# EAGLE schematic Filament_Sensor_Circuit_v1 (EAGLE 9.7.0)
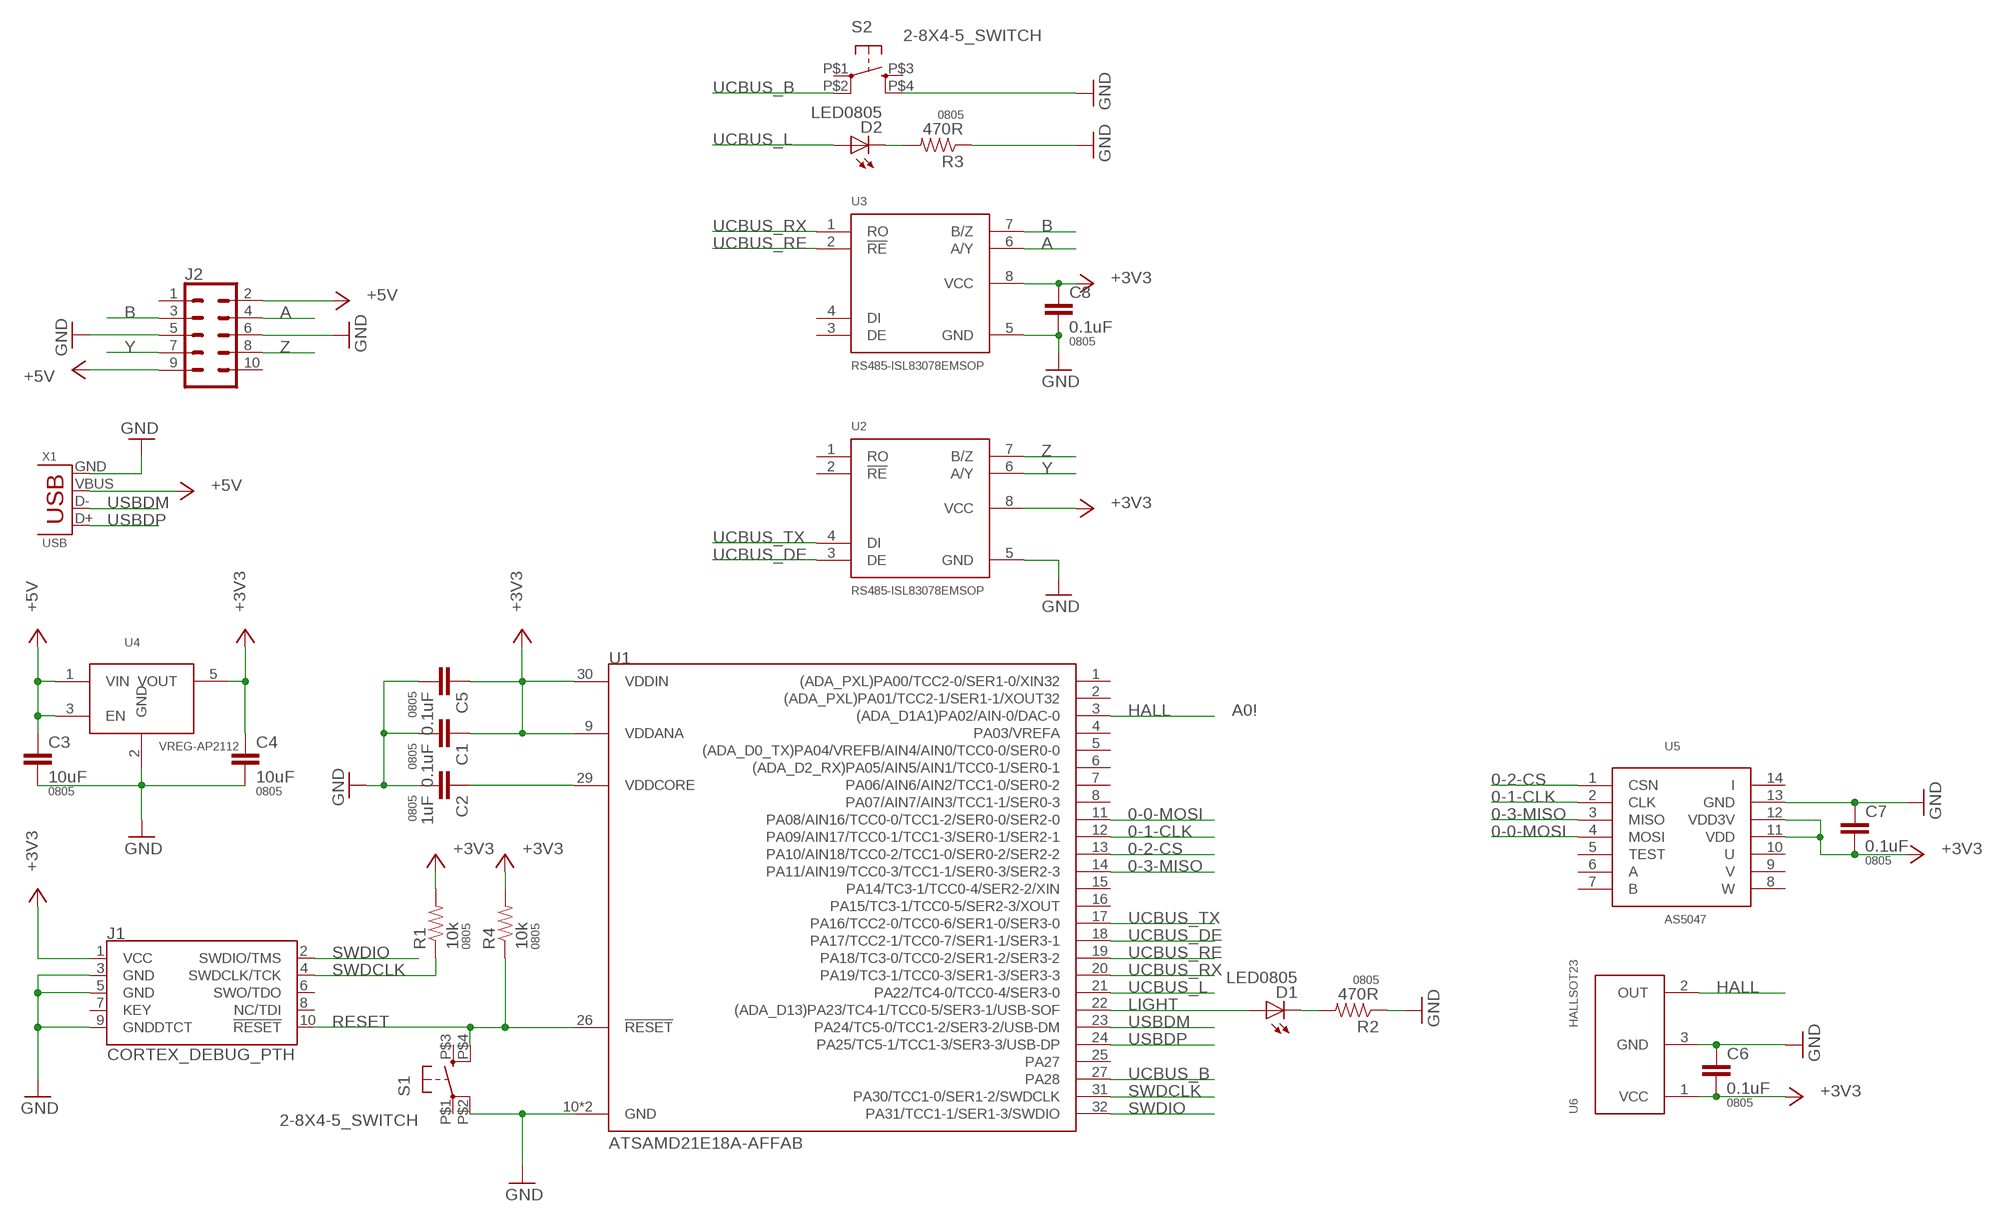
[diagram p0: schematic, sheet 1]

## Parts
C1  0.1uF  CAP0805  [0805]
C2  1uF  CAP0805  [0805]
C3  10uF  CAP0805  [0805]
C4  10uF  CAP0805  [0805]
C5  0.1uF  CAP0805  [0805]
C6  0.1uF  CAP0805  [0805]
C7  0.1uF  CAP0805  [0805]
C8  0.1uF  CAP0805  [0805]
D1  LED0805  [LED0805]
D2  LED0805  [LED0805]
J1  CORTEX_DEBUG_PTH  [2X5-PTH-1.27MM]
J2  CONN_05X2SHD_LOCK_LATCH  [2X5-SHROUDED_LOCK_LATCH]
R1  10k  RESISTOR0805-RES  [0805]
R2  470R  RESISTOR0805-RES  [0805]
R3  470R  RESISTOR0805-RES  [0805]
R4  10k  RESISTOR0805-RES  [0805]
S1  2-8X4-5_SWITCH  [TACT-SWITCH-KMR6]
S2  2-8X4-5_SWITCH  [TACT-SWITCH-KMR6]
U1  ATSAMD21E18A-AFFAB  [TQFP-32-FAB]
U2  RS485-ISL83078EMSOP  [8-MSOP]
U3  RS485-ISL83078EMSOP  [8-MSOP]
U4  VREG-AP2112  [SOT23-5]
U5  AS5047  [TSSOP14]
U6  HALLSOT23  [SOT23]
X1  USB  [USB_MICRO_609-4613-1-ND]

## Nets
0-0-MOSI: U1.11(PA08/AIN16/TCC0-0/TCC1-2/SER0-0/SER2-0) U5.4(MOSI)
0-1-CLK: U1.12(PA09/AIN17/TCC0-1/TCC1-3/SER0-1/SER2-1) U5.2(CLK)
0-2-CS: U1.13(PA10/AIN18/TCC0-2/TCC1-0/SER0-2/SER2-2) U5.1(CSN)
0-3-MISO: U1.14(PA11/AIN19/TCC0-3/TCC1-1/SER0-3/SER2-3) U5.3(MISO)
+3V3: C1.1 C4.1 C5.1 C6.2 C7.2 C8.1 J1.1(VCC) R1.2 R4.2 U1.9(VDDANA) U1.30(VDDIN) U2.8(VCC) U3.8(VCC) U4.5(VOUT) U5.11(VDD) U5.12(VDD3V) U6.1(VCC)
+5V: C3.1 J2.2 J2.9 U4.1(VIN) U4.3(EN) X1.VBUS
A: J2.4 U3.6(A/Y)
B: J2.3 U3.7(B/Z)
GND: C1.2 C2.2 C3.2 C4.2 C5.2 C6.1 C7.1 C8.2 J1.3(GND) J1.5(GND) J1.9(GNDDTCT) J2.5 J2.6 R2.1 R3.1 S1.P$2(P1) S2.P$4(S1) U1.10(GND) U1.28(GND) U2.5(GND) U3.5(GND) U4.2(GND) U5.13(GND) U6.3(GND) X1.GND
HALL: U1.3((ADA_D1A1)PA02/AIN-0/DAC-0) U6.2(OUT)
LIGHT: D1.1(A) U1.22((ADA_D13)PA23/TC4-1/TCC0-5/SER3-1/USB-SOF)
N$1: D1.2(C) R2.2
N$2: D2.2(C) R3.2
N$5: C2.1 U1.29(VDDCORE)
RESET: J1.10(!RESET) R4.1 S1.P$4(S1) U1.26(!RESET)
SWDCLK: J1.4(SWDCLK/TCK) R1.1 U1.31(PA30/TCC1-0/SER1-2/SWDCLK)
SWDIO: J1.2(SWDIO/TMS) U1.32(PA31/TCC1-1/SER1-3/SWDIO)
UCBUS_B: S2.P$2(P1) U1.27(PA28)
UCBUS_DE: U1.18(PA17/TCC2-1/TCC0-7/SER1-1/SER3-1) U2.3(DE)
UCBUS_L: D2.1(A) U1.21(PA22/TC4-0/TCC0-4/SER3-0)
UCBUS_RE: U1.19(PA18/TC3-0/TCC0-2/SER1-2/SER3-2) U3.2(!RE)
UCBUS_RX: U1.20(PA19/TC3-1/TCC0-3/SER1-3/SER3-3) U3.1(RO)
UCBUS_TX: U1.17(PA16/TCC2-0/TCC0-6/SER1-0/SER3-0) U2.4(DI)
USBDM: U1.23(PA24/TC5-0/TCC1-2/SER3-2/USB-DM) X1.D-
USBDP: U1.24(PA25/TC5-1/TCC1-3/SER3-3/USB-DP) X1.D+
Y: J2.7 U2.6(A/Y)
Z: J2.8 U2.7(B/Z)
Unconnected: J1.6(SWO/TDO) J1.7(KEY) J1.8(NC/TDI) J2.1 J2.10 S1.P$1(P) S1.P$3(S) S2.P$1(P) S2.P$3(S) U1.1((ADA_PXL)PA00/TCC2-0/SER1-0/XIN32) U1.2((ADA_PXL)PA01/TCC2-1/SER1-1/XOUT32) U1.4(PA03/VREFA) U1.5((ADA_D0_TX)PA04/VREFB/AIN4/AIN0/TCC0-0/SER0-0) U1.6((ADA_D2_RX)PA05/AIN5/AIN1/TCC0-1/SER0-1) U1.7(PA06/AIN6/AIN2/TCC1-0/SER0-2) U1.8(PA07/AIN7/AIN3/TCC1-1/SER0-3) U1.15(PA14/TC3-1/TCC0-4/SER2-2/XIN) U1.16(PA15/TC3-1/TCC0-5/SER2-3/XOUT) U1.25(PA27) U2.1(RO) U2.2(!RE) U3.3(DE) U3.4(DI) U5.5(TEST) U5.6(A) U5.7(B) U5.8(W) U5.9(V) U5.10(U) U5.14(I)

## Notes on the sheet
- A0!

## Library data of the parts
C1-C8 = passives:CAP: Capacitor; PACKAGE: 0805
D1 D2 = lights:LED: LED
J1 = SparkFun-Connectors:CORTEX_DEBUG: Cortex Debug Connector - 10 pin Supports JTAG debug, Serial Wire debug, and Serial Wire Viewer. PTH and SMD connector options available. General Connector Information Products: PTH Connector -via Digi-Key SparkFun PSoc SparkFun T
J2 = SparkFun-Connectors:CONN_05X2: Multi connection point. Often used as Generic Header-pin footprint for 0.1 inch spaced/style header connections For AVR SPI programming port, see special device with nice symbol: "AVR_SPI_PROG_5x2.dev" You can populate with any combo of single row headers, but if you'd like an exact match, check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
R1-R4 = passives:RESISTOR: Resistor; PACKAGE: 0805
S1 S2 = passives:2-8X4-5_SWITCH
U1 = microcontrollers:ATSAMD21E18A-AF: The SAM D21 is a series of low-power microcontrollers using the 32-bit ARM® Cortex® -M0+ processor, and ranging from 32- to 64-pins with up to 256KB Flash and 32KB of SRAM. The SAM D21 operate at a maximum frequency of 48MHz and reach 2.46 CoreMark® /MHz. Check prices
U2 U3 = comm:RS485-ISL83078E
U4 = power:VREG-AP2112
U5 = sensor:AS5047
U6 = sensor:HALL
X1 = connector:USB: SMD micro USB connector as found in the fablab inventory. Three footprint variants included: 609-4613-1-ND used by Jake original, as described by manufacturer's datasheet for milling with the 1/100" bit for milling with the 1/64" bit Made by Zaerc.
